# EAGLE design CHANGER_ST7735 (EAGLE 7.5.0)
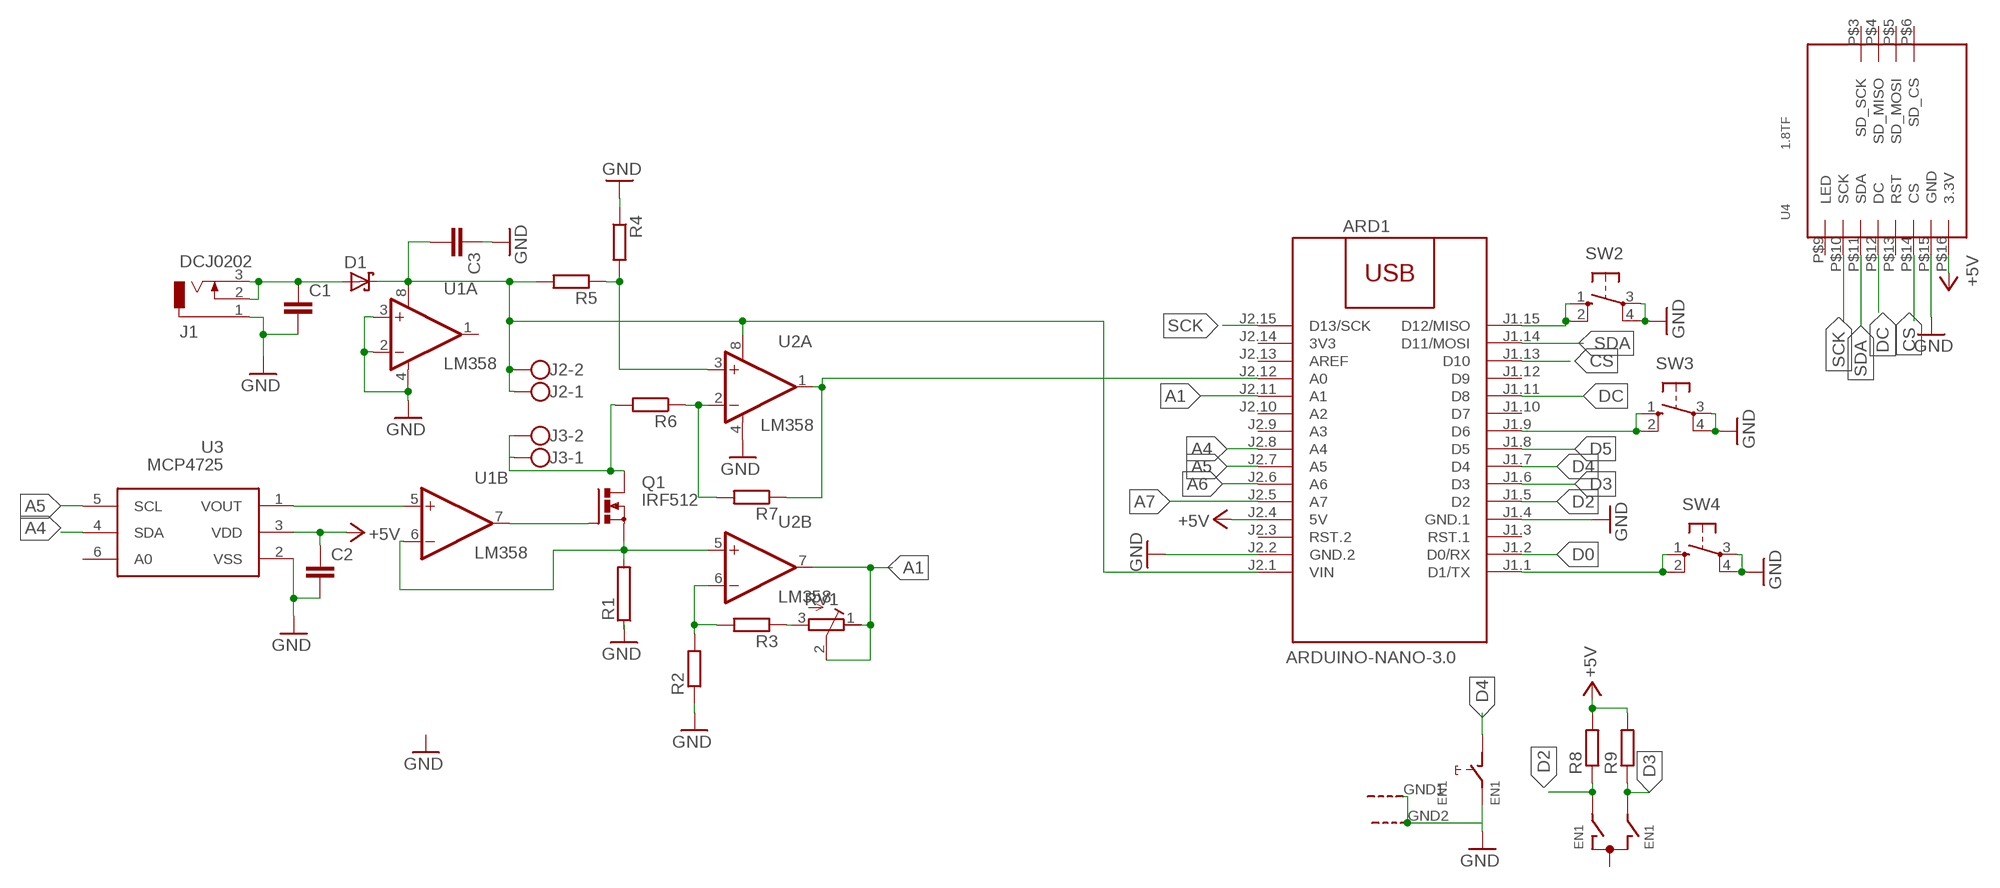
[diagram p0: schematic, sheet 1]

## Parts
ARD1  ARDUINO-NANO-3.0  [ARDUINO-NANO-3.0]
C1  C-EUC1206  [C1206]
C2  C-EUC1206  [C1206]
C3  C-EUC1206  [C1206]
D1  MBR1560  [TO220ACS]
EN1  EN1  EC12E_SW  [ALPS_EC12E_SW]
J1  DCJ0202  [DCJ0202]
J2  W237-102  [W237-102]
J3  W237-102  [W237-102]
Q1  IRF512  [TO220BV]
R1  RAC04  [AC04]
R2  R-EU_R1206  [R1206]
R3  R-EU_R1206  [R1206]
R4  R-EU_R1206  [R1206]
R5  R-EU_R1206  [R1206]
R6  R-EU_R1206  [R1206]
R7  R-EU_R1206  [R1206]
R8  R-EU_R1206  [R1206]
R9  R-EU_R1206  [R1206]
RV1  R-TRIMM-3386-F  [R-TRIMM-3386F]
SW2  10-XX  [B3F-10XX]
SW3  10-XX  [B3F-10XX]
SW4  10-XX  [B3F-10XX]
U1  LM358  OPA2650P  [DIL08]
U2  LM358  OPA2650P  [DIL08]
U3  MCP4725  [SOT23-6]
U4  1.8TF  [1.8TFT]

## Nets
+5V: ARD1.J2.4(5V) C2.1 R8.2 R9.2 U3.3(VDD) U4.P$16(3.3V)
A1: ARD1.J2.11(A1) RV1.1(A) RV1.2(S) U2.7(B:OUT)
A4: ARD1.J2.8(A4) U3.4(SDA)
A5: ARD1.J2.7(A5) U3.5(SCL)
A6: ARD1.J2.6(A6)
A7: ARD1.J2.5(A7)
CS: ARD1.J1.13(D10) U4.P$14(CS)
D0: ARD1.J1.2(D0/RX)
D2: ARD1.J1.5(D2) EN1.A R8.1
D3: ARD1.J1.6(D3) EN1.B R9.1
D4: ARD1.J1.7(D4) EN1.D
D5: ARD1.J1.8(D5)
DC: ARD1.J1.11(D8) U4.P$12(DC)
GND: ARD1.J1.4(GND.1) ARD1.J2.2(GND.2) C1.2 C2.2 C3.1 EN1.E EN1.GND1(G) EN1.GND2(G) J1.1 R1.1 R2.1 R4.1 SW2.3(P) SW2.4(P1) SW3.3(P) SW3.4(P1) SW4.3(P) SW4.4(P1) U1.2(A:-IN) U1.3(A:+IN) U1.4(A:V-) U2.4(A:V-) U3.2(VSS) U4.P$15(GND)
N$1: U1.5(B:+IN) U3.1(VOUT)
N$2: Q1.G U1.7(B:OUT)
N$3: ARD1.J1.9(D6) SW3.1(S) SW3.2(S1)
N$4: ARD1.J1.1(D1/TX) SW4.1(S) SW4.2(S1)
N$7: C1.1 D1.A J1.2 J1.3
N$17: ARD1.J1.15(D12/MISO) SW2.1(S) SW2.2(S1)
N$33: Q1.S R1.2 U1.6(B:-IN) U2.5(B:+IN)
N$34: J3.1 J3.2 Q1.D R6.2
N$35: R3.1 RV1.3(E)
N$36: R2.2 R3.2 U2.6(B:-IN)
N$37: R4.2 R5.1 U2.3(A:+IN)
N$38: R6.1 R7.2 U2.2(A:-IN)
N$39: ARD1.J2.12(A0) R7.1 U2.1(A:OUT)
SCK: ARD1.J2.15(D13/SCK) U4.P$10(SCK)
SDA: ARD1.J1.14(D11/MOSI) U4.P$11(SDA)
VIN1: ARD1.J2.1(VIN) C3.2 D1.C J2.1 J2.2 R5.2 U1.8(A:V+) U2.8(A:V+)
Unconnected: ARD1.J1.3(RST.1) ARD1.J1.10(D7) ARD1.J1.12(D9) ARD1.J2.3(RST.2) ARD1.J2.9(A3) ARD1.J2.10(A2) ARD1.J2.13(AREF) EN1.C U1.1(A:OUT) U3.6(A0) U4.P$3(SD_SCK) U4.P$4(SD_MISO) U4.P$5(SD_MOSI) U4.P$6(SD_CS) U4.P$9(LED) U4.P$13(RST)

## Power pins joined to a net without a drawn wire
3V3: ARD1.J2.14(3V3)

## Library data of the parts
ARD1 = diy-modules:ARDUINO-NANO-3.0: Arduino Nano 3.0 and compatible devices More details available here: https://www.arduino.cc/en/Main/ArduinoBoardNano Click here to find device on ebay.com
C1-C3 = rcl:C-EU: CAPACITOR, European symbol
D1 = diode:MBR1560
EN1 = switch-alps:EC12E_SW: ALPS rotary Encoder EC12E series with switch; MPN: EC12E2424407; OC_FARNELL: 1520813; OC_NEWARK: 74M1068
J1 = con-jack:DCJ0202: DC POWER JACK Source: DCJ0202.pdf; OC_FARNELL: unknown; OC_NEWARK: unknown
J2 J3 = con-wago-500:W237-102: WAGO SCREW CLAMP; MPN: 237-102; OC_FARNELL: unknown; OC_NEWARK: 70K9898
Q1 = transistor-power:IRF512: N-CHANNEL MOS FET
R1 = resistor-power:R: Power Resitor; OC_FARNELL: unknown; OC_NEWARK: unknown
R2-R9 = rcl:R-EU_: RESISTOR, European symbol
RV1 = rcl:R-TRIMM-3386-F
SW2-SW4 = switch-omron:10-XX: OMRON SWITCH; MPN: B3F-1000; OC_FARNELL: 176432; OC_NEWARK: 36M3542
U1 U2 = burr-brown:OPA2650: Dual Wideband, Low Power Voltage Feedback Operational Amplifier; MPN: AD8056ANZ; OC_FARNELL: 1079308; OC_NEWARK: 19M0925
U3 = linear:MCP4725
U4 = tft_1_8_1_44_oled_0_96:1.8TF

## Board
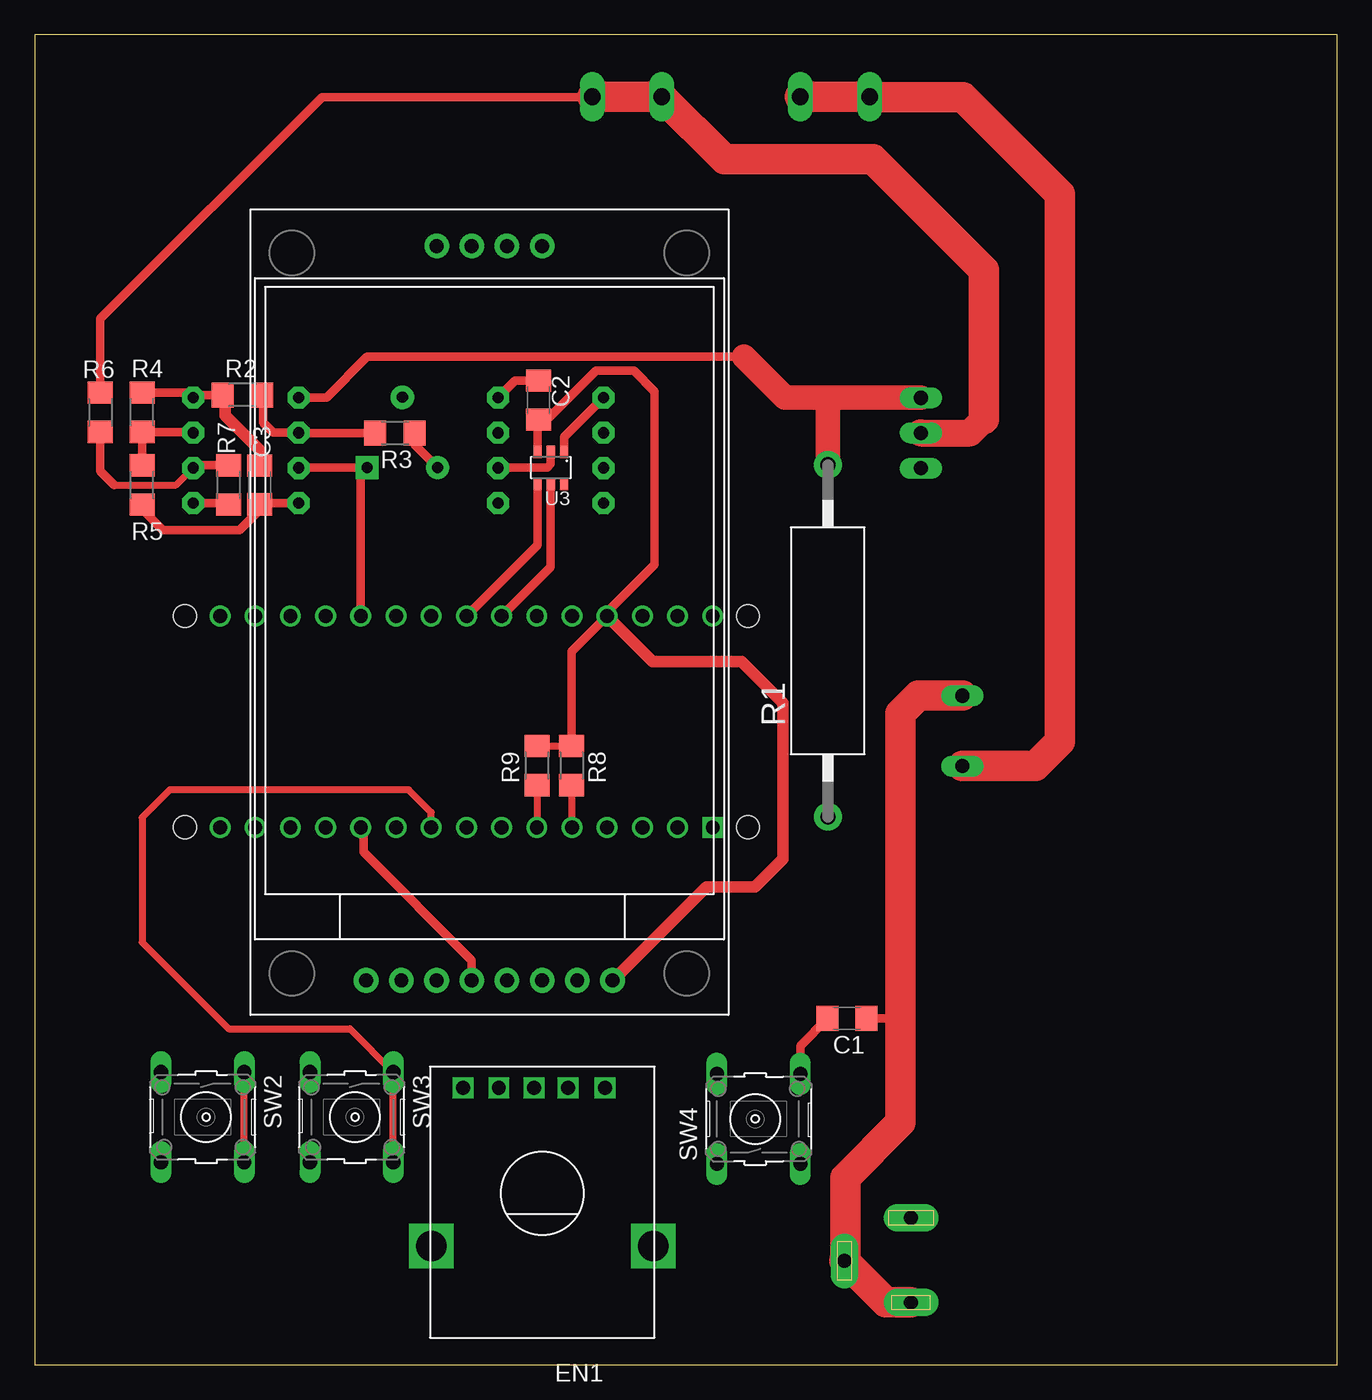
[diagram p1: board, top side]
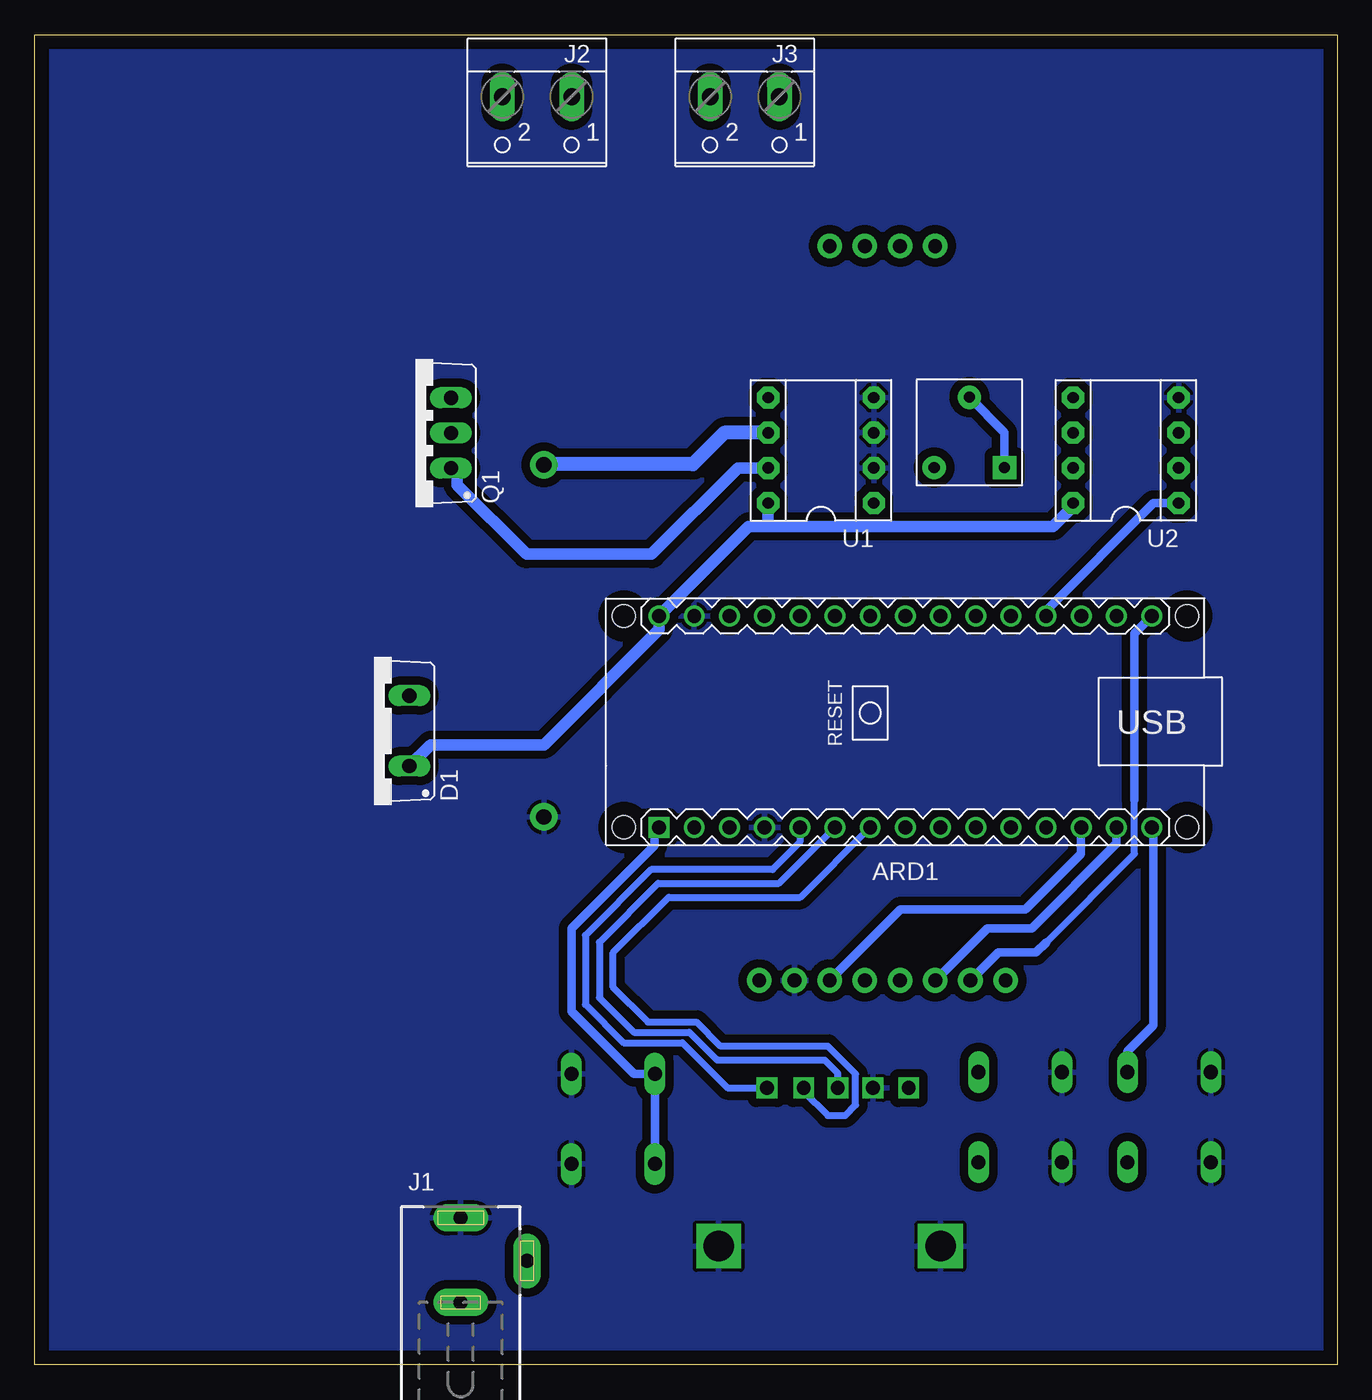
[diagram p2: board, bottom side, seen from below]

Size 94 x 96 mm. Coordinates in mm from the lower left corner, seen from the top.
Outline: 0,0 94,0 94,96 0,96 0,0
Copper layers (1*16): Top 0.035mm / dielectric 1.5mm / Bottom 0.035mm
Design rules "default": minimum track width 10mil, minimum drill 24mil, track to track 8mil, track to pad 8mil, pad to pad 8mil, via to via 8mil, smd to smd 8mil, copper to edge 40mil, drill to drill 8mil, minimum pad ring 10mil, minimum via ring 8mil, stop-mask expansion 4mil, vias tented up to drill 0mil, thermal gap 10mil

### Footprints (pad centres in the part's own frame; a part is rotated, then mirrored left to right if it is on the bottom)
ARDUINO-NANO-3.0 = drill 1 square: J1.1 17.78,7.62 | drill 1: J1.2 15.24,7.62; J1.3 12.7,7.62; J1.4 10.16,7.62; J1.5 7.62,7.62; J1.6 5.08,7.62; J1.7 2.54,7.62; J1.8 0,7.62; J1.9 -2.54,7.62; J1.10 -5.08,7.62; J1.11 -7.62,7.62; J1.12 -10.16,7.62; J1.13 -12.7,7.62; J1.14 -15.24,7.62; J1.15 -17.78,7.62; J2.1 17.78,-7.62; J2.2 15.24,-7.62; J2.3 12.7,-7.62; J2.4 10.16,-7.62; J2.5 7.62,-7.62; J2.6 5.08,-7.62; J2.7 2.54,-7.62; J2.8 0,-7.62; J2.9 -2.54,-7.62; J2.10 -5.08,-7.62; J2.11 -7.62,-7.62; J2.12 -10.16,-7.62; J2.13 -12.7,-7.62; J2.14 -15.24,-7.62; J2.15 -17.78,-7.62 | hole 1.651: -20.32,7.62; -20.32,-7.62; 20.32,-7.62; 20.32,7.62
C1206 = smd 1.6 x 1.8: 1 -1.4,0; 2 1.4,0
TO220ACS = drill 1.016 long: A 2.54,-2.54; C -2.54,-2.54
ALPS_EC12E_SW = drill 1 square: A 5.16,7.605; B 0.04,7.605; C -5.08,7.605; D 2.5,7.605; E -2.5,7.605 | drill 2.2 square: GND1 8.64,-3.81; GND2 -7.37,-3.81
DCJ0202 = drill 1 pad 2 long: 1 0,3.1; 2 4.8,0; 3 0,-3
W237-102 = drill 1.194 long: 1 -2.5,-1.27; 2 2.5,-1.27
TO220BV = drill 1.016 long: D 0,-2.54; G -2.54,-2.54; S 2.54,-2.54
AC04 = drill 1.1 pad 2: 1 -12.7,0; 2 12.7,0
R1206 = smd 1.6 x 1.803: 1 -1.422,0; 2 1.422,0
R-TRIMM-3386F = drill 0.8 pad 1.676 square: 1 0,0 | drill 0.8 pad 1.676: 2 5.08,2.54; 3 0,5.08
B3F-10XX = drill 1.016 long: 1 -3.251,2.761; 2 3.251,2.761; 3 -3.251,-3.261; 4 3.251,-3.261
DIL08 = drill 0.813 pad 1.6 octagon: 1 -3.81,-3.81; 2 -1.27,-3.81; 3 1.27,-3.81; 4 3.81,-3.81; 5 3.81,3.81; 6 1.27,3.81; 7 -1.27,3.81; 8 -3.81,3.81
SOT23-6 = smd 0.6 x 0.9: 1 -0.95,-1.15; 2 0,-1.15; 3 0.95,-1.15; 4 0.95,1.15; 5 0,1.15; 6 -0.95,1.15
1.8TFT = drill 1 pad 1.778: P$3 55.5,21.05; P$4 55.5,18.52; P$5 55.5,15.98; P$6 55.5,13.44; P$9 2.5,26.14; P$10 2.5,23.6; P$11 2.5,21.06; P$12 2.5,18.52; P$13 2.5,15.98; P$14 2.5,13.44; P$15 2.5,10.9; P$16 2.5,8.36

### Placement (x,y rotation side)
ARD1  31.16,46.41 180 bottom
C1  58.62,25 180 top
C2  36.38,69.62 90 top
C3  16.25,63.5 270 top
D1  69.5,45.75 90 bottom
EN1  36,12.38 0 top
J1  63.25,7.5 0 bottom
J2  57.75,90.25 180 bottom
J3  42.75,90.25 180 bottom
Q1  66.5,67.25 90 bottom
R1  57.25,52.25 90 top
R2  15,70 0 top
R3  26,67.25 180 top
R4  7.75,68.75 270 top
R5  7.75,63.5 270 top
R6  4.75,68.75 90 top
R7  14,63.5 90 top
R8  38.75,43.25 90 top
R9  36.25,43.25 90 top
RV1  24,64.75 90 bottom
SW2  12.38,17.88 270 top
SW3  23.12,17.88 270 top
SW4  52,17.75 90 top
U1  37.25,66 90 bottom
U2  15.25,66 90 bottom
U3  37.25,64.75 180 top
U4  50.06,25.25 90 top

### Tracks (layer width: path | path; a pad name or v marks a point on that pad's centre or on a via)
+5V
  Top 0.5: R9.2 R8.2
  Top 0.61: U3.3 36.3,68.15 C2.1 36.4,68.25 37,68.25 40.5,71.75 43.25,71.75 44.75,70.25 44.75,57.75 41.32,54.32 ARD1.J2.4 38.75,51.47 R8.2
  Top 0.813: 41.32,53.68 ARD1.J2.4 44.6,50.75 51,50.75 54,47.75 54,36.5 52,34.5 48.5,34.5 41.74,27.75 U4.P$16
A1
  Top 0.61: U2.7 19.08,64.75 RV1.1 23.54,64.29 ARD1.J2.11
  Bottom 0.61: RV1.1 24,67.29 RV1.2
A4
  Top 0.61: U3.4 36.3,59.17 ARD1.J2.8
A5
  Top 0.61: U3.5 37.25,57.59 ARD1.J2.7
CS
  Bottom 0.61: U4.P$14 31.5,32.88 22.5,32.88 18.5,36.88 18.5,38.76 ARD1.J1.13
D2
  Top 0.5: R8.1 38.75,38.83 ARD1.J1.5
  Bottom 0.5: ARD1.J1.5 38.78,37.72 40.75,35.75 49.5,35.75 54.25,31 54.25,26 51.5,23.25 47.25,23.25 44,20 41.18,20 EN1.A
D3
  Top 0.5: R9.1 ARD1.J1.6
  Bottom 0.5: EN1.B 36.04,21.04 37,22 44.75,22 46.75,24 50.75,24 53.25,26.5 53.25,30.5 49,34.75 40.28,34.75 ARD1.J1.6
D4
  Bottom 0.5: EN1.D 38.5,19.75 36.75,18 35.5,18 34.75,18.75 34.75,21 36.75,23 44.5,23 46.25,24.75 49.75,24.75 52.25,27.25 52.25,29.75 48.25,33.75 38.75,33.75 ARD1.J1.7
DC
  Top 0.61: U4.P$12 31.55,29.2 23.75,37 23.75,38.59 ARD1.J1.11
GND
  Top 0.61: R4.1 11.08,70.17 U2.4 11.63,70 R2.1 | C3.1 16.25,65 | C2.2 34.66,71.03 U1.4 | U3.2 37.25,65 37,64.75 33.46,64.75 U1.2 | SW4.4 55.26,23.04 C1.2
  Top 0.813: 16.25,65 16.25,66 13.75,68.5 13.75,69.83 R2.1
  pour Bottom (isolate 0.61): 0.75,95.5 92.75,95.5 92.75,0.25 0.75,0.25
N$1
  Top 0.61: U3.1 38.2,66.95 U1.5
N$2
  Bottom 0.813: U1.7 43.25,64.73 49.48,58.5 58.5,58.5 63.5,63.5 63.5,64.25 Q1.G
N$3
  Top 0.5: ARD1.J1.9 28.62,39.88 27,41.5 9.75,41.5 7.75,39.5 7.75,30.5 14,24.25 22.76,24.25 SW3.1 SW3.2
N$4
  Bottom 0.61: SW4.1 SW4.2 50.75,21 55.25,25.5 55.25,31.5 49.25,37.5 49.25,38.48 ARD1.J1.1
N$7
  Top 0.61: C1.1 62.5,25
  Top 2.184: D1.A 63.79,48.29 62.5,47 62.5,25 62.5,17.5 58.5,13.5 58.5,7.55 J1.2 61.45,4.5 J1.3
N$17
  Top 0.5: SW2.2 SW2.1
  Bottom 0.61: SW2.1 15.14,22.61 13.25,24.5 13.25,38.66 ARD1.J1.15
N$33
  Top 0.61: U2.5 21.06,69.81 24,72.75 51.2,72.75
  Top 1.778: Q1.S 57,69.79 | 57,69.79 54.16,69.79 51.2,72.75 | R1.2 57.25,69.54 57,69.79
  Bottom 1.016: U1.6 44.23,67.27 46.5,65 57.2,65 R1.2
N$34
  Top 0.61: R6.2 4.75,75.5 20.75,91.5 40.23,91.5 J3.1
  Top 1.93: Q1.D 67.5,67.25 68.5,68.25
  Top 2.184: J3.1 J3.2 49.77,87 60.5,87 68.5,79 68.5,68.25
N$35
  Top 0.61: R3.1 27.42,66.41 RV1.3
N$36
  Top 0.61: R2.2 16.5,69.92 16.5,68 17.23,67.27 U2.6 19.08,67.25 R3.2
N$37
  Top 0.61: R5.1 R4.2 11.38,67.33 U2.3
N$38
  Top 0.5: 5.75,63.5 10.21,63.5 U2.2
  Top 0.61: R7.2 11.63,64.92 U2.2 | R6.1 4.75,64.5 5.75,63.5
N$39
  Top 0.61: U2.1 13.89,62.19 R7.1
  Bottom 0.61: ARD1.J2.12 21,54.44 13.25,62.19 U2.1
SCK
  Bottom 0.5: 21,30.5 14.62,36.88 14.62,40.75
  Bottom 0.61: 14.62,40.75 14.62,52.79 ARD1.J2.15 | 21,30.5 21.75,29.75 24.46,29.75 U4.P$10
SDA
  Bottom 0.61: ARD1.J1.14 15.92,37.62 22.05,31.5 25.25,31.5 U4.P$11
VIN1
  Top 0.61: U2.8 16.75,62.19 | 16.75,62.19 16.34,62.19 C3.2 | R5.2 7.75,61.75 9.25,60.25 14.81,60.25 16.75,62.19
  Top 2.184: D1.C 72.21,43.21 74,45 74,84.5 67,91.5 60.27,91.5 J2.2 J2.1
  Bottom 0.61: U2.8 19.06,61.94
  Bottom 0.813: 19.06,61.94 20.5,60.5 41,60.5 | 41,60.5 42.48,60.5 ARD1.J2.1 48.94,53.06 57.25,44.75 65.42,44.75 D1.C | U1.8 41.06,60.56 41,60.5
